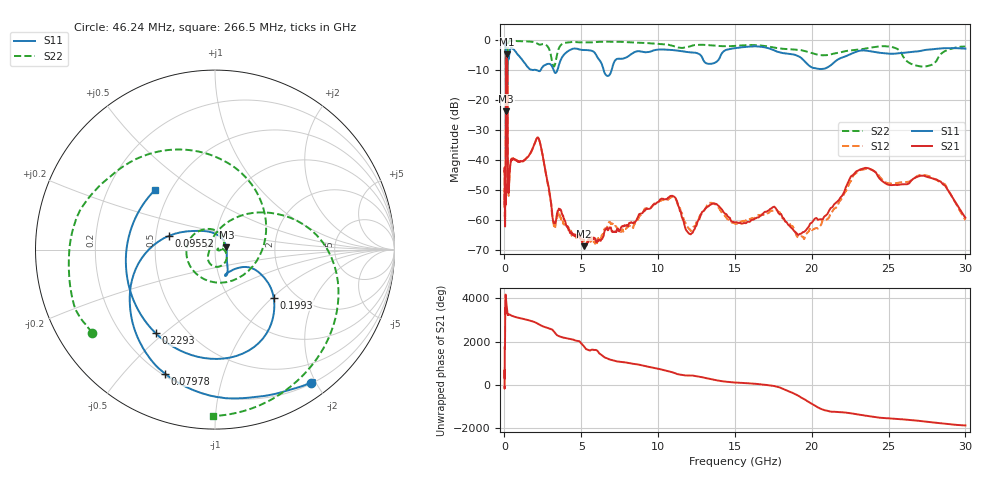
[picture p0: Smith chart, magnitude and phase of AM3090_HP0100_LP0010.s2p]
! Date/Time: Thu, Feb 28, 2019 1:57 PM
! Network Analyzer: Agilent Technologies E8364B Rev: A.07.50.67
! Sweep from 0.010 to 30.000 GHz, 1601 Points, Sweep Type: LOG
! Power Supply: 5.023 V, 0.002 A
# Hz S DB R 50
!freq MagS11 AngS11 MagS21 AngS21 MagS12 AngS12 MagS22 AngS22
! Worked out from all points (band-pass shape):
!   1601 points, 10 MHz to 30 GHz, reference 50 ohm
!   highest |S21| = -4.76 dB at 141.8 MHz (marker M1); lowest = -68.8 dB at 5.18 GHz (marker M2)
!   |S21| within 3 dB of the highest: 104.6 MHz to 184.5 MHz (79.95 MHz wide, 55.3 % of centre)
!   lowest |S11| = -23.8 dB at 103.5 MHz (marker M3), VSWR 1.14, Z = 56.7 + j1.46 ohm
!   |S11| at or under -10 dB: 2.051 GHz to 2.361 GHz (309.8 MHz wide, 14 % of centre); 3.198 GHz to 3.452 GHz (253.9 MHz wide, 7.64 % of centre); 6.454 GHz to 6.979 GHz (524.2 MHz wide, 7.8 % of centre)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
!   |S22| runs from -37.9 to -0.2 dB; largest |S21 - S12| = 0.013
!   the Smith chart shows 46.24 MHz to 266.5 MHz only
!   S11 on the Smith chart (normalised r, x): 46.24 MHz: 0.21, -1.94; 79.78 MHz: 0.21, -0.65; 95.52 MHz: 0.59, +0.10; 199.3 MHz: 1.57, -1.02; 229.3 MHz: 0.34, -0.47; 266.5 MHz: 0.41, +0.35
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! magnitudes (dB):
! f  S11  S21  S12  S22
! 10 MHz  -0.2  -43.9  -44.1  -0.5
! 38.04 MHz  -0.5  -58.5  -59.9  -1.3
! 46.24 MHz  -0.8  -51.2  -49.9  -1.7
! 79.78 MHz  -2.6  -47.4  -46.5  -5.3
! 95.52 MHz  -11.5  -15.4  -15.4  -14.9
! 103.5 MHz  -23.8  -8.2  -8.2  -16.7
! 130.3 MHz  -16.3  -4.9  -4.9  -37.8
! 141.8 MHz  -16.7  -4.8  -4.7  -26.0
! 144.7 MHz  -16.7  -4.8  -4.7  -23.6
! 177.7 MHz  -14.5  -6.5  -6.5  -30.6
! 199.3 MHz  -7.5  -17.4  -17.4  -10.0
! 229.3 MHz  -4.9  -50.6  -50.8  -1.5
! 266.5 MHz  -6.5  -50.2  -51.3  -0.6
! 550.5 MHz  -3.0  -39.7  -39.6  -0.3
! 2.084 GHz  -10.0  -33.0  -33.0  -1.0
! 3.204 GHz  -10.1  -60.8  -61.3  -8.9
! 5.18 GHz  -3.4  -68.8  -67.1  -0.8
! 7.926 GHz  -5.8  -62.0  -62.8  -0.7
! 10.7 GHz  -3.3  -52.6  -53.0  -1.6
! 19.7 GHz  -8.0  -62.9  -64.4  -3.9
! 23.59 GHz  -3.6  -42.7  -43.1  -2.7
! 30 GHz  -2.9  -59.3  -60.1  -2.2
